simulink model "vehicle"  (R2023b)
settings: Solver=ode3  StartTime=0.0  StopTime=t_end  FixedStep=dt8dof  RelTol=1e-3
PreLoadFcn:
  | define_swarm_buses(3, 1000);
model workspace (MAT data in the model file):
  Af = 1.8
  Cp_tyre = 500
  Cx = 0.28
  G = 15000
  Ha = 0.4
  Hg = 0.4
  Hroll = 0.304
  Hroll_f = 0.08
  Hroll_r = 0.12
  Ir = 0.8
  Ix = 450
  Jz = 1800
  K = 130000
  K_psi = 0.48
  K_y = 0.06
  Karb_F = 26000
  Karb_R = 26000
  KdF = 0
  KdR = 0
  Kd_h = 0
  Kd_v = 0
  Kd_y = 0
  Ki_h = 0
  Ki_v = 0.1
  Ki_y = 0
  Kp_h = 1.5
  Kp_v = 1.5
  Kp_y = 0.1
  Ks_f = 39000
  Ks_r = 39000
  Kv = 290000
  L = 1.5
  Lril_L = 0.055
  Lril_T = 0.5
  MAX_PATH_LEN = 1000
  Pacn = [3000 1 1 1 1 1 1 1 1 0 0 0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]
  R0 = 0.2
  Rfront = 0.2
  Rr_sterzo = 0
  Rrear = 0.2
  Rs = 13
  Tf = 1.5
  Tr = 1.5
  a = 0.6
  a_brake = -3
  b = 0.9
  camb_0F = 0
  camb_0R = -0.00680678408278
  d_max = 0.558505360638
  dt8dof = 0.002
  dtastar = 0.1
  dtcontrol = 0.03
  f0 = 0.0041
  f2 = 2.051e-07
  g = 9.81
  m = 1300
  mot_T_table = [0 0 0 0 0 0 0 0 0 0 0 0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]
  mot_alpha_bp = [0 10 20 30 40 50 60 70 80 90 100]
  mot_n_bp = [0 29.9163426864 59.8326853729 89.7490280593 119.665370746 149.581713432 179.498056119 209.414398805 239.330741492 269.247084178 299.163426864 329.079769551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]
  mpc_speed : object (value not decoded)
  phi_road0 = 0
  psi0 = 0
  r_goal = 5
  r_slow = 30
  replan_steps = 20
  rho = 1.3
  slope_x_body0 = 0
  slope_y_body0 = 0
  t_end = 70
  terrain_truth_mu_table = [-1 -1 -1 -1 -1 -1 -1 -1 -1 -1 -1 -1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]
  terrain_truth_obstacle_table = [1 1 1 1 1 1 1 1 1 1 1 1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]
  terrain_truth_slope_deg_table = [2.67415653197 2.67413215857 2.67406695826 2.6739952249 2.6739164067 2.67382991742 2.67373513563 2.67363140411 2.67351802953 2.67339428225 2.67325939642 2.67311257041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]
  terrain_truth_slope_x_table = [-0.0458815772305 -0.0458808922252 -0.0458794511544 -0.0458778616187 -0.0458761104845 -0.0458741837099 -0.0458720663111 -0.0458697423295 -0.0458671948025 -0.0458644057365 -0.0458613560839 -0.045858025724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]
  terrain_truth_slope_y_table = [0.00874081815183 0.00874213563744 0.00874360556 0.00874524373283 0.00874706738108 0.00874909524079 0.00875134766185 0.00875384671474 0.00875661630067 0.00875968226488 0.00876307251276 0.0087668171283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]
  terrain_truth_traversable_table = [0 0 0 0 0 0 0 0 0 0 0 0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]
  terrain_truth_x_bp = [0 1 2 3 4 5 6 7 8 9 10 11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]
  terrain_truth_y_bp = [0 1 2 3 4 5 6 7 8 9 10 11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]
  teta0 = 0
  tetapunto0 = 0
  theta_road0 = 0
  toe_F = -0.00174532925199
  toe_R = 0.00174532925199
  velstart = 5
  wr0_FL = 3.15
  wr0_FR = 3.15
  wr0_RL = 3.15
  wr0_RR = 3.15
  x0 = 0
  y0 = 0
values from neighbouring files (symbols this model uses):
  gear_ratio = 10    [motor_map.m]
  v_ref_init = scenario.vehicle8.velstart    [make_vref_filter.m]
undefined symbols (not defined in the file or in its folder): A_f, B_f, C_f, D_f, psi0_1
libraries: simulink_extras x15, mpclib x1, slpidlib x1
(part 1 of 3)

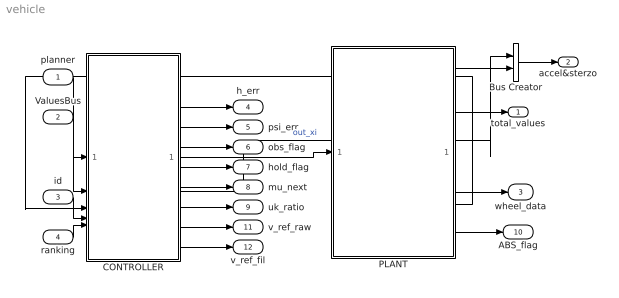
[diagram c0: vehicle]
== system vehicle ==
  planner : Inport  OutDataTypeStr=Bus: PlannerPath  SampleTime=.1
  ValuesBus : Inport  Port=2  OutDataTypeStr=Bus: ValuesBus
  id : Inport  Port=3
  ranking : Inport  Port=4  PortDimensions=3
  Bus Creator : BusCreator  Inputs=2  OutDataTypeStr=Bus: AccelSterzo
  CONTROLLER : Subsystem
  PLANT : Subsystem
  total_values : Outport  OutDataTypeStr=Bus: VehicleState
  accel&sterzo : Outport  Port=2  OutDataTypeStr=Bus: AccelSterzo
  wheel_data : Outport  Port=3  OutDataTypeStr=Bus: WheelData
  h_err : Outport  Port=4
  psi_err : Outport  Port=5
  obs_flag : Outport  Port=6
  hold_flag : Outport  Port=7
  mu_next : Outport  Port=8
  uk_ratio : Outport  Port=9
  ABS_flag : Outport  Port=10
  v_ref_raw : Outport  Port=11
  v_ref_fil : Outport  Port=12
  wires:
  PLANT/1(Out_delta) -> Bus Creator/2
  CONTROLLER/2(Out_xi) -> Bus Creator/1  "out_xi"
  planner/1 -> CONTROLLER/1(from planner)
  CONTROLLER/1(to_plant) -> PLANT/1(from_controller)
  Bus Creator/1 -> accel&sterzo/1
  PLANT/2(total_values) -> total_values/1
  PLANT/3(to_controller) -> CONTROLLER/3(from_plant)
  id/1 -> CONTROLLER/4(id)
  ranking/1 -> CONTROLLER/5(ranking)
  ValuesBus/1 -> CONTROLLER/2(ValuesBus)
  PLANT/4(wheel_data) -> wheel_data/1
  CONTROLLER/3(e_cte) -> h_err/1
  CONTROLLER/4(psi_e) -> psi_err/1
  CONTROLLER/5(obs_flag) -> obs_flag/1
  CONTROLLER/6(hold_flag) -> hold_flag/1
  CONTROLLER/7(mu next) -> mu_next/1
  CONTROLLER/8(unk_ratio) -> uk_ratio/1
  PLANT/5(ABS_flag) -> ABS_flag/1
  CONTROLLER/9(v_ref_raw) -> v_ref_raw/1
  CONTROLLER/10(v_ref_fil) -> v_ref_fil/1

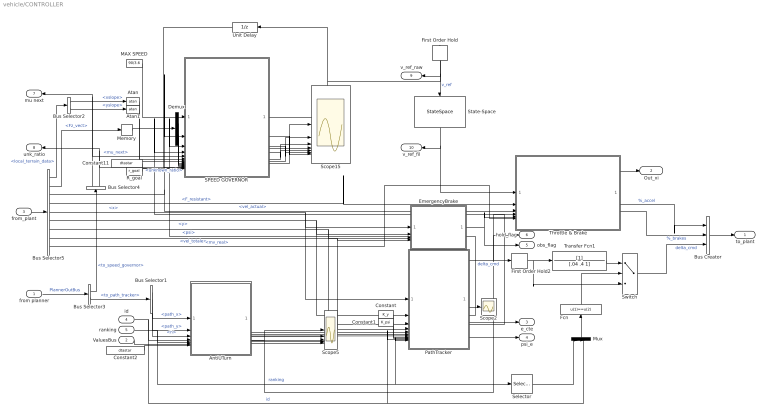
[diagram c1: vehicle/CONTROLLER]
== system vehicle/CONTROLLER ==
  from planner : Inport
  ValuesBus : Inport  Port=2
  from_plant : Inport  Port=3
  id : Inport  Port=4
  ranking : Inport  Port=5
  AntiUTurn : MATLAB Function  TreatAsAtomicUnit=on
  Atan : Trigonometry  Operator=atan
  Atan1 : Trigonometry  Operator=atan
  Bus Creator : BusCreator  Inputs=3
  Bus Selector1 : BusSelector  OutputSignals=path_x,path_y,n
  Bus Selector2 : BusSelector  OutputSignals=slope_vehicle.xslope,slope_vehicle.yslope
  Bus Selector3 : BusSelector  OutputSignals=to_speed_governor,to_path_tracker
  Bus Selector4 : BusSelector  OutputSignals=mu_next,unknown_ratio
  Bus Selector5 : BusSelector  OutputSignals=local_terrain_data,Fz_vect,vel_actual,F_resistant,signal2.x,signal2.y,signal2.psi,signal2.vel_totale,mv_real
  Constant : Constant  Value=K_y
  Constant1 : Constant  Value=K_psi
  Constant11 : Constant  Value=dtastar
  Constant2 : Constant  Value=dtastar
  Demux : Demux
  EmergencyBrake : MATLAB Function  TreatAsAtomicUnit=on
  Fcn : Fcn  Expr=u(1)==u(2)
  First Order Hold : FirstOrderHold  InitialOutput=v_ref_init  ErrorTolerance=inf
  First Order Hold2 : FirstOrderHold  ErrorTolerance=inf
  MAX SPEED : Constant  Value=90/3.6
  Memory : Memory
  Mux : Mux  Inputs=2
  PathTracker : MATLAB Function  TreatAsAtomicUnit=on
  R_goal : Constant  Value=r_goal
  SPEED GOVERNOR : MATLAB Function  TreatAsAtomicUnit=on
  Scope15 : Scope  NumInputPorts=7
  Scope2 : Scope
  Scope5 : Scope  NumInputPorts=5
  Selector : Selector  InputPortWidth=3  IndexOptions=Index vector (dialog)  Indices=[1]  OutputSizes=1
  State-Space : StateSpace  A=A_f  B=B_f  C=C_f  D=D_f  InitialCondition=v_ref_init
  Switch : Switch  Criteria=u2 > Threshold
  Throttle & Brake : Subsystem
  Transfer Fcn1 : TransferFcn  Denominator=[.04 .4 1]
  Unit Delay : UnitDelay  InitialCondition=velstart  SampleTime=-1  HasFrameUpgradeWarning=on
  to_plant : Outport
  Out_xi : Outport  Port=2
  e_cte : Outport  Port=3
  psi_e : Outport  Port=4
  obs_flag : Outport  Port=5
  hold_flag : Outport  Port=6
  mu next : Outport  Port=7
  unk_ratio : Outport  Port=8
  v_ref_raw : Outport  Port=9
  v_ref_fil : Outport  Port=10
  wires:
  Constant11/1 -> SPEED GOVERNOR/14(Ts)
  PathTracker/6(psi_e) -> psi_e/1
  PathTracker/3(dist_to_goal) -> SPEED GOVERNOR/4(d_goal)
  MAX SPEED/1 -> SPEED GOVERNOR/1("v_max_global ")
  Bus Selector4/1 -> SPEED GOVERNOR/5(mu_next), mu next/1  "<mu_next>"
  SPEED GOVERNOR/2(v_ref_raw) -> Scope15/1
  Bus Selector3/1 -> Bus Selector4/1  "<to_speed_governor>"
  from planner/1 -> Bus Selector3/1  "PlannerOutBus"
  PathTracker/2(kappa_next) -> SPEED GOVERNOR/3(kappa_next)
  Bus Selector5/6 -> PathTracker/2(y), EmergencyBrake/2(y)  "<y>"
  PathTracker/1(delta_cmd) -> First Order Hold2/1  "delta_cmd"
  Bus Selector5/5 -> PathTracker/1(x), EmergencyBrake/1(x)  "<x>"
  Bus Selector5/7 -> PathTracker/3(psi), EmergencyBrake/3(psi)  "<psi>"
  SPEED GOVERNOR/7(v_unknown) -> Scope15/6
  PathTracker/4(goal_flag) -> Scope2/1
  SPEED GOVERNOR/8(v_ltr) -> Scope15/7
  First Order Hold/1 -> State-Space/1, v_ref_raw/1  "v_ref"
  SPEED GOVERNOR/4(v_curve_mu) -> Scope15/3
  Bus Selector2/2 -> Atan1/1  "<yslope>"
  SPEED GOVERNOR/1(v_ref) -> First Order Hold/1, Unit Delay/1
  Memory/1 -> Demux/1
  Atan1/1 -> SPEED GOVERNOR/7(angle_lat)
  SPEED GOVERNOR/3(v_max_global) -> Scope15/2
  Bus Selector2/1 -> Atan/1  "<xslope>"
  Demux/3 -> SPEED GOVERNOR/10(Fz_RL)
  SPEED GOVERNOR/6(v_goal) -> Scope15/5
  Bus Selector4/2 -> SPEED GOVERNOR/12(unknown_ratio_ahead), unk_ratio/1  "<unknown_ratio>"
  SPEED GOVERNOR/5(v_rollover) -> Scope15/4
  Atan/1 -> SPEED GOVERNOR/6(angle_long)
  Demux/1 -> SPEED GOVERNOR/8(Fz_FL)
  Bus Selector3/2 -> Bus Selector1/1  "<to_path_tracker>"
  Demux/2 -> SPEED GOVERNOR/9(Fz_FR)
  R_goal/1 -> SPEED GOVERNOR/15(r_goal)
  Demux/4 -> SPEED GOVERNOR/11(Fz_RR)
  Constant/1 -> PathTracker/8(K_y)
  Constant1/1 -> PathTracker/9(K_psi)
  Bus Creator/1 -> to_plant/1
  from_plant/1 -> Bus Selector5/1
  Bus Selector5/3 -> SPEED GOVERNOR/2(V), Throttle & Brake/3(v_actual)  "<vel_actual>"
  Bus Selector5/1 -> Bus Selector2/1  "<local_terrain_data>"
  Bus Selector5/2 -> Memory/1  "<Fz_vect>"
  Throttle & Brake/2(% accel) -> Bus Creator/1  "%_accel"
  Throttle & Brake/3(brakes) -> Bus Creator/2  "%_brakes"
  Throttle & Brake/1(Out_xi) -> Out_xi/1
  Bus Selector5/4 -> Throttle & Brake/2(F_res)  "<F_resistant>"
  Bus Selector5/8 -> PathTracker/4(vel), EmergencyBrake/4(vel)  "<vel_totale>"
  First Order Hold2/1 -> Transfer Fcn1/1, Switch/3
  AntiUTurn/1(path_x_out) -> PathTracker/5(path_x)
  AntiUTurn/2(path_y_out) -> PathTracker/6(path_y)
  AntiUTurn/3(n_out) -> PathTracker/7(n_pts)
  Bus Selector1/1 -> AntiUTurn/1(path_x_in)  "<path_x>"
  Bus Selector1/2 -> AntiUTurn/2(path_y_in)  "<path_y>"
  Bus Selector1/3 -> AntiUTurn/3(n_in)  "<n>"
  id/1 -> AntiUTurn/4(id), Mux/2, PathTracker/10(id)  "id"
  ranking/1 -> Selector/1, PathTracker/11(ranking), AntiUTurn/5(ranking)  "ranking"
  ValuesBus/1 -> AntiUTurn/6(ValuesBus)
  Constant2/1 -> AntiUTurn/7(Ts)
  AntiUTurn/4(hold_flag) -> Scope5/1, hold_flag/1, Throttle & Brake/4(hold_flag)
  AntiUTurn/5(allow_uturn) -> Scope5/2
  AntiUTurn/6(long_rel) -> Scope5/3
  AntiUTurn/7(wait_s) -> Scope5/4
  AntiUTurn/8(mode) -> Scope5/5
  EmergencyBrake/1(obs_flag) -> obs_flag/1, Throttle & Brake/5(emergency_flag)
  Unit Delay/1 -> SPEED GOVERNOR/13(v_ref_prev)
  State-Space/1 -> Throttle & Brake/1(v_ref), v_ref_fil/1
  PathTracker/5(e_cte) -> e_cte/1
  Switch/1 -> Bus Creator/3  "delta_cmd"
  Selector/1 -> Mux/1
  Mux/1 -> Fcn/1
  Fcn/1 -> Switch/2
  Transfer Fcn1/1 -> Switch/1
  Bus Selector5/9 -> Throttle & Brake/6(mv_real)  "<mv_real>"

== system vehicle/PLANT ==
  note: questi sono i plot degli slip, far vedere come si notano i diversi sample time: ogni .1 cambia il comando motore e lo slip torna ad oscillare, ma grazie alle lunghezze di rilassamento (che rendono stiff il problema) lo slip si smorza intorno al valore
  from_controller : Inport
  Bus Creator : BusCreator  Inputs=6
  Bus Selector : BusSelector  OutputSignals=delta_cmd,%_accel,%_brakes
  ENGINE : Subsystem
  Gain : Gain  Gain=-1
  Rate Limiter delta : RateLimiter  RisingSlewLimit=1.5  FallingSlewLimit=-1.5  SampleTimeMode=inherited
  Sat_delta : Saturate  UpperLimit=d_max  LowerLimit=-d_max
  VEHICLE 8DOF : Subsystem
  get_values : Subsystem
  Out_delta : Outport
  total_values : Outport  Port=2
  to_controller : Outport  Port=3
  wheel_data : Outport  Port=4
  ABS_flag : Outport  Port=5
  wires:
  get_values/3(local terrain data) -> Bus Creator/6, VEHICLE 8DOF/4(terrain)  "local_terrain_data"
  VEHICLE 8DOF/3(speed_vel) -> get_values/1(speed_vel)
  get_values/1(total_values) -> total_values/1, Bus Creator/2
  ENGINE/1(Cm_vect) -> VEHICLE 8DOF/2(Cm_vect)
  Rate Limiter delta/1 -> Out_delta/1, VEHICLE 8DOF/1(delta)  "delta_sterzo"
  Sat_delta/1 -> Rate Limiter delta/1
  get_values/2(vel_actual) -> Bus Creator/3  "vel_actual"
  Gain/1 -> Sat_delta/1
  VEHICLE 8DOF/2(Fz_vect) -> Bus Creator/1  "Fz_vect"
  from_controller/1 -> Bus Selector/1
  Bus Selector/1 -> Gain/1  "<delta_cmd>"
  Bus Creator/1 -> to_controller/1
  Bus Selector/2 -> ENGINE/2(% accel)  "<%_accel>"
  Bus Selector/3 -> VEHICLE 8DOF/3(%brakes)  "<%_brakes>"
  VEHICLE 8DOF/4(F_res) -> Bus Creator/4  "F_resistant"
  VEHICLE 8DOF/1(wheel_data) -> wheel_data/1, ENGINE/1(wheel_data)
  VEHICLE 8DOF/5(ABS_flag) -> ABS_flag/1
  VEHICLE 8DOF/6(mv_real) -> Bus Creator/5  "mv_real"

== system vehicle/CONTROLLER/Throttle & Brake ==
  v_ref : Inport
  F_res : Inport  Port=2
  v_actual : Inport  Port=3
  hold_flag : Inport  Port=4
  emergency_flag : Inport  Port=5
  mv_real : Inport  Port=6
  Abs : Abs
  Add : Sum
  Const_zero_alpha : Constant  Value=0
  Constant : Constant  Value=0
  Constant1 : Constant  Value=-400
  MATLAB Function : MATLAB Function  TreatAsAtomicUnit=on
  MPC Controller : mpclib/MPC Controller  SCDEnableBlockLinearizationSpecification=on  mpcobj=mpc_speed  is_multiple=0  enable_value=0  return_u0=off  updateMPCinCallerWorkspace=on  md_inport=on  mv_inport=on  uref_inport=off  return_cost=off  return_mvseq=off  return_qpstatus=off  return_xseq=off  return_state=off  return_ovseq=off  state_inport=off  umin_inport=off  umax_inport=off  ymin_inport=off  ymax_inport=on  cc_inport=off  ywt_inport=off  uwt_inport=off  duwt_inport=off  rhoeps_inport=off  pm_inport=off  MaximumP=20  HorizonChoice=FixedHorizon  n_ts=0.03  n_p=30  n_mv=1  n_md=1  n_ud=0  n_mo=1  n_uo=0  BlockDataType=double  SampleTimeInherited=off  switch_inport=off
  Max_alpha_pos : MinMax  Function=max  Inputs=2
  Min : MinMax  Inputs=2
  Switch : Switch  Criteria=u2 > Threshold
  Switch1 : Switch  Criteria=u2 > Threshold
  Switch2 : Switch  Criteria=u2 > Threshold
  Unit Delay : UnitDelay  SampleTime=-1  HasFrameUpgradeWarning=on
  Zero-Order Hold : ZeroOrderHold  SampleTime=dt8dof
  Out_xi : Outport
  % accel : Outport  Port=2
  brakes : Outport  Port=3
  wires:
  Zero-Order Hold/1 -> Min/1, Max_alpha_pos/1
  v_ref/1 -> MPC Controller/2, MPC Controller/5
  v_actual/1 -> MPC Controller/1, MATLAB Function/1(v_actual)
  Max_alpha_pos/1 -> Switch/3  "% accel"
  Const_zero_alpha/1 -> Min/2, Max_alpha_pos/2
  hold_flag/1 -> Add/2
  Constant/1 -> Switch/1
  Switch/1 -> Switch2/2, Switch2/1, % accel/1
  Add/1 -> Switch/2
  emergency_flag/1 -> Switch1/2, Add/1
  Constant1/1 -> Switch1/1
  Min/1 -> Switch1/3
  Switch1/1 -> Switch2/3, Abs/1
  Switch2/1 -> Unit Delay/1, Out_xi/1
  Abs/1 -> brakes/1
  MPC Controller/1 -> Zero-Order Hold/1
  F_res/1 -> MATLAB Function/3(F_res)
  Unit Delay/1 -> MATLAB Function/2(accel_prev)
  MATLAB Function/1(F_md) -> MPC Controller/3
  mv_real/1 -> MPC Controller/4

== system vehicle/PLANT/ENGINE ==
  wheel_data : Inport
  % accel : Inport  Port=2
  Apply_factor : Product  Inputs=**
  Bus Selector1 : BusSelector  OutputSignals=w_r_vect,slip_vect
  Gain_gear : Gain  Gain=gear_ratio
  Gain_n2 : Gain  Gain=gear_ratio*60/(2*pi)
  Motor_Map4 : Lookup_n-D  BreakpointsForDimension1=mot_n_bp  BreakpointsForDimension2=mot_alpha_bp  BreakpointsForDimension3=[5, 7]  Table=mot_T_table  ExtrapMethod=Clip  InternalRulePriority=Speed  RndMeth=Simplest
  TC_PI : slpidlib/PID Controller  Controller=PI  Form=Parallel  TimeDomain=Continuous-time  UseExternalTs=off  SampleTime=-1  IntegratorMethod=Forward Euler  FilterMethod=Forward Euler  ControllerParametersSource=internal  P=4  I=15  UseKiTs=off  D=0  N=100  UseFilter=on  TunerSelectOption=Transfer Function Based (PID Tuner App)  InitialConditionSource=internal  InitialConditionForIntegrator=1  InitialConditionForFilter=0  DifferentiatorICPrevScaledInput=0  ExternalReset=none  TrackingMode=off  Kt=1  LimitOutput=on  SatLimitsSource=internal  UpperSaturationLimit=1  LowerSaturationLimit=0  LinearizeAsGain=on  AntiWindupMode=clamping  Kb=1  LimitIntegrator=off  UpperIntegratorSaturationLimit=inf  LowerIntegratorSaturationLimit=-inf  POutMin=[]  POutMax=[]  IOutMin=[]  IOutMax=[]  DOutMin=[]  DOutMax=[]  NOutMin=[]  NOutMax=[]  SumOutMin=[]  SumOutMax=[]  SaturationOutMin=[]  SaturationOutMax=[]  PParamMin=[]  PParamMax=[]  IParamMin=[]  IParamMax=[]  DParamMin=[]  DParamMax=[]  NParamMin=[]  NParamMax=[]  KbParamMin=[]  KbParamMax=[]  KtParamMin=[]  KtParamMax=[]  KbOutMin=[]  KbOutMax=[]  KtOutMin=[]  KtOutMax=[]  IntegratorOutMin=[]  IntegratorOutMax=[]  FilterOutMin=[]  FilterOutMax=[]  SumI1OutMin=[]  SumI1OutMax=[]  SumI2OutMin=[]  SumI2OutMax=[]  SumI3OutMin=[]  SumI3OutMax=[]  SumI4OutMin=[]  SumI4OutMax=[]  SumDOutMin=[]  SumDOutMax=[]  DifferentiatorOutMin=[]  DifferentiatorOutMax=[]  FilterDiffOutCoefMin=[]  FilterDiffOutCoefMax=[]  ReciprocalOutMin=[]  ReciprocalOutMax=[]  SumDenOutMin=[]  SumDenOutMax=[]  SumNumOutMin=[]  SumNumOutMax=[]  DivideOutMin=[]  DivideOutMax=[]  UdiffTsProdOutMin=[]  UdiffTsProdOutMax=[]  NTsProdOutMin=[]  NTsProdOutMax=[]  UintegralTsProdOutMin=[]  UintegralTsProdOutMax=[]  UngainTsProdOutMin=[]  UngainTsProdOutMax=[]  ClampingZeroOutDataTypeStr=Inherit: Inherit via back propagation  ClampingZeroOutMin=[]  ClampingZeroOutMax=[]  FilterDenConstantOutDataTypeStr=Inherit: Inherit via back propagation  FilterDenConstantOutMin=[]  FilterDenConstantOutMax=[]  PCopyOutDataTypeStr=Inherit: Inherit via back propagation  PCopyOutMin=[]  PCopyOutMax=[]  NCopyOutDataTypeStr=Inherit: Inherit via back propagation  NCopyOutMin=[]  NCopyOutMax=[]  IntegratorContinuousStateAttributes=''  IntegratorStateMustResolveToSignalObject=off  IntegratorRTWStateStorageClass=Auto  FilterContinuousStateAttributes=''  FilterStateMustResolveToSignalObject=off  FilterRTWStateStorageClass=Auto  ParallelPVariant=InternalParameters  IdealPVariant=Disabled  IVariant=InternalParameters  DVariant=Disabled  IntegratorVariant=Continuous  SatVariant=Enabled  AWVariant=ContClampingParallel  PCopyVariant=Disabled  TRVariant=Disabled  FdbkBlocksVariant=Forward  IdealPFdbkVariant=Disabled  SatFdbkVariant=Disabled  DerivativeFilterVariant=Disabled  NVariant=Disabled  NCopyVariant=Disabled_SignalSpec  FilterICVariant=Disabled  IntegratorICVariant=InternalICs  ExternalResetVariant=Disabled  TRSumVariant=Passthrough  SumFdbkVariant=Disabled  SumVariant=Sum_PI  TsampFilterVariant=InternalTs  TsampNgainVariant=Passthrough  TsampIntegralVariant=Disabled_SignalSpec  ExternalSaturationOutDataTypeStr=Inherit: Same as second input
  alpha_sat : Saturate  UpperLimit=100  LowerLimit=0
  sigma_star : Constant  Value=0.10
  slip_err : Sum  Inputs=+-
  Cm_vect : Outport
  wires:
  wheel_data/1 -> Bus Selector1/1
  alpha_sat/1 -> Motor_Map4/2
  TC_PI/1 -> Apply_factor/2
  sigma_star/1 -> slip_err/1
  Apply_factor/1 -> alpha_sat/1
  Bus Selector1/1 -> Gain_n2/1  "<w_r_vect>"
  Bus Selector1/2 -> slip_err/2  "<slip_vect>"
  Gain_gear/1 -> Cm_vect/1
  slip_err/1 -> TC_PI/1
  Gain_n2/1 -> Motor_Map4/1
  Motor_Map4/1 -> Gain_gear/1
  % accel/1 -> Apply_factor/1

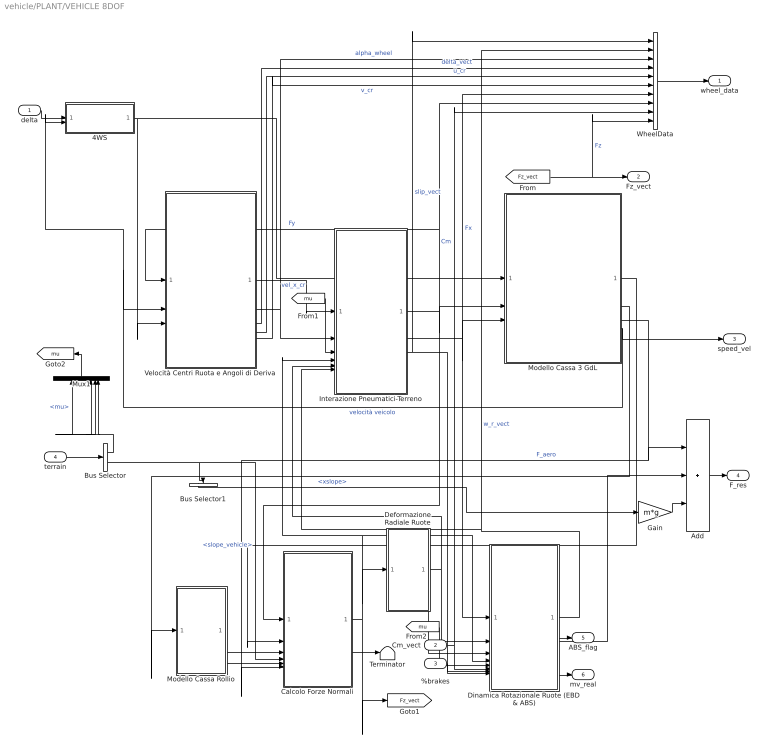
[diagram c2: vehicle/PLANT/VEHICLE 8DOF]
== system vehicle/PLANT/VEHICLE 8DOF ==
  delta : Inport
  Cm_vect : Inport  Port=2
  %brakes : Inport  Port=3
  terrain : Inport  Port=4
  4WS : Subsystem
  Add : Sum  Inputs=+++
  Bus Selector : BusSelector  OutputSignals=mu,slope_vehicle
  Bus Selector1 : BusSelector  OutputSignals=xslope
  Calcolo Forze Normali : Subsystem
  Deformazione Radiale Ruote : Subsystem
  Dinamica Rotazionale Ruote (EBD & ABS) : Subsystem
  Gain : Gain  Gain=m*g
  Interazione Pneumatici-Terreno : Subsystem
  Modello Cassa 3 GdL : Subsystem
  Modello Cassa Rollio : Subsystem
  Mux1 : Mux
  Terminator : Terminator
  Velocità Centri Ruota e Angoli di Deriva : Subsystem
  WheelData : BusCreator  Inputs=10
  wheel_data : Outport  VectorParamsAs1DForOutWhenUnconnected=off
  Fz_vect : Outport  Port=2
  speed_vel : Outport  Port=3
  F_res : Outport  Port=4  VectorParamsAs1DForOutWhenUnconnected=off
  ABS_flag : Outport  Port=5  VectorParamsAs1DForOutWhenUnconnected=off
  mv_real : Outport  Port=6  VectorParamsAs1DForOutWhenUnconnected=off
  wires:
  Interazione Pneumatici-Terreno/1(Fy) -> Calcolo Forze Normali/1(Fy), Modello Cassa 3 GdL/2(Fy), WheelData/8, Velocità Centri Ruota e Angoli di Deriva/1(Fy)  "Fy"
  [mu] -> Interazione Pneumatici-Terreno/3(mu)
  Interazione Pneumatici-Terreno/2(Fx) -> Modello Cassa 3 GdL/3(Fx), Dinamica Rotazionale Ruote (EBD & ABS)/1(Fx), WheelData/7  "Fx"
  Velocità Centri Ruota e Angoli di Deriva/2(alpha) -> Interazione Pneumatici-Terreno/2(alpha), WheelData/3  "alpha_wheel"
  Dinamica Rotazionale Ruote (EBD & ABS)/1(w_r) -> Interazione Pneumatici-Terreno/6(w_r), WheelData/2  "w_r_vect"
  Deformazione Radiale Ruote/1(Rr) -> Dinamica Rotazionale Ruote (EBD & ABS)/2(Rr), Interazione Pneumatici-Terreno/5(Rr)
  Deformazione Radiale Ruote/2(Rc) -> Dinamica Rotazionale Ruote (EBD & ABS)/3(Rc)
  Modello Cassa 3 GdL/3(F_aero) -> Calcolo Forze Normali/6(Faero), Add/1  "F_aero"
  Calcolo Forze Normali/2("FzF/FzR ") -> Terminator/1
  %brakes/1 -> Dinamica Rotazionale Ruote (EBD & ABS)/7(%brakes)
  Mux1/1 -> [mu]
  Modello Cassa 3 GdL/2(a_y) -> Modello Cassa Rollio/1(acc_y)
  Cm_vect/1 -> Dinamica Rotazionale Ruote (EBD & ABS)/6(Cm), WheelData/9  "Cm"
  Velocità Centri Ruota e Angoli di Deriva/1(vel_x_cr) -> Interazione Pneumatici-Terreno/1(vel_x_cr)  "vel_x_cr"
  Modello Cassa Rollio/1(phi_punto) -> Calcolo Forze Normali/3(phi_punto)
  Modello Cassa 3 GdL/1(a_x) -> Calcolo Forze Normali/2(acc_x)
  Modello Cassa Rollio/2(phi) -> Calcolo Forze Normali/5(phi)
  Interazione Pneumatici-Terreno/3(slip_vector) -> Dinamica Rotazionale Ruote (EBD & ABS)/8(slip_vect), WheelData/1  "slip_vect"
  terrain/1 -> Bus Selector/1
  Bus Selector/1 -> Mux1/1, Mux1/2, Mux1/3, Mux1/4  "<mu>"
  Bus Selector/2 -> Bus Selector1/1, Calcolo Forze Normali/4(slope)  "<slope_vehicle>"
  Modello Cassa 3 GdL/4(velocità_veicolo) -> speed_vel/1, 4WS/2(velocità_veicolo), Velocità Centri Ruota e Angoli di Deriva/2(velocità_veicolo)  "velocità veicolo"
  4WS/1(delta_ruote) -> Modello Cassa 3 GdL/1(delta_cmd), Velocità Centri Ruota e Angoli di Deriva/3(delta_cmd)
  delta/1 -> 4WS/1(delta_sterzo)
  WheelData/1 -> wheel_data/1
  Calcolo Forze Normali/1(Fz) -> Deformazione Radiale Ruote/1(Fz), Dinamica Rotazionale Ruote (EBD & ABS)/4(Fz), Interazione Pneumatici-Terreno/4(Fz), [Fz_vect]
  Dinamica Rotazionale Ruote (EBD & ABS)/2(R_roll_tot) -> Add/2
  Add/1 -> F_res/1
  Gain/1 -> Add/3
  Bus Selector1/1 -> Gain/1  "<xslope>"
  [mu] -> Dinamica Rotazionale Ruote (EBD & ABS)/5(mu)
  Velocità Centri Ruota e Angoli di Deriva/3(delta_vect) -> WheelData/4  "delta_vect"
  Velocità Centri Ruota e Angoli di Deriva/4(u_cr) -> WheelData/5  "u_cr"
  Velocità Centri Ruota e Angoli di Deriva/5(v_cr) -> WheelData/6  "v_cr"
  [Fz_vect] -> WheelData/10, Fz_vect/1  "Fz"
  Dinamica Rotazionale Ruote (EBD & ABS)/3(ABS_flag) -> ABS_flag/1
  Dinamica Rotazionale Ruote (EBD & ABS)/4(mv_real) -> mv_real/1

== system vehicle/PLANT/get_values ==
  speed_vel : Inport
  Bus Creator2 : BusCreator  Inputs=4
  Bus Selector : BusSelector  OutputSignals=uv
  Constant5 : Constant  Value=x0
  Constant6 : Constant  Value=y0
  Integrator : Integrator  InitialConditionSource=external
  Integrator1 : Integrator  InitialConditionSource=external
  Lookup Tables : Subsystem
  Pitagora : Subsystem
  rotazione : Subsystem
  total_values : Outport
  vel_actual : Outport  Port=2
  local terrain data : Outport  Port=3
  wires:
  Integrator/1 -> Lookup Tables/1(x), Bus Creator2/1  "x"
  Constant5/1 -> Integrator/2
  Constant6/1 -> Integrator1/2
  rotazione/1(x_dot) -> Integrator/1
  Integrator1/1 -> Lookup Tables/2(y), Bus Creator2/2  "y"
  rotazione/2(y_dot) -> Integrator1/1
  Pitagora/1(vel_actual) -> Bus Creator2/4, vel_actual/1  "vel_totale"
  Lookup Tables/1(data) -> local terrain data/1
  speed_vel/1 -> Bus Selector/1, rotazione/1(velocità_veicolo)
  Bus Selector/1 -> Pitagora/1(u_v)  "<uv>"
  rotazione/3(psi) -> Lookup Tables/3(psi), Bus Creator2/3  "psi"
  Bus Creator2/1 -> total_values/1

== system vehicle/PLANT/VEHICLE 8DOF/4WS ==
  delta_sterzo : Inport
  velocità_veicolo : Inport  Port=2
  100km/h : Constant  Value=28
  Bus Creator : BusCreator  Inputs=2
  Bus Selector : BusSelector  OutputSignals=uv.u
  Constant : Constant
  Divide : Product  Inputs=**
  Divide1 : Product  Inputs=*/
  Divide2 : Product  Inputs=**
  Fcn : Fcn  Expr=1/(1+exp(-(u(1)-u(2))/2.22))
  Fcn1 : Fcn  Expr=u(3)+u(1)*(u(2)-u(3))
  Gain2 : Gain  Gain=.3
  K2_high : Constant  Value=.3
  K2_low : Constant  Value=-.4
  Min : MinMax  Inputs=2
  Minus : Sum  Inputs=-+
  Mux : Mux  Inputs=2
  Mux1 : Mux  Inputs=3
  vel_transizione : Constant  Value=10
  delta_ruote : Outport
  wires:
  Divide1/1 -> Min/1
  velocità_veicolo/1 -> Bus Selector/1
  100km/h/1 -> Divide1/2
  Bus Selector/1 -> Divide1/1, Mux/1  "<u>"
  Min/1 -> Gain2/1
  vel_transizione/1 -> Mux/2
  Constant/1 -> Minus/2, Min/2
  Mux/1 -> Fcn/1
  Fcn/1 -> Mux1/1  "sigmoide"
  K2_high/1 -> Mux1/2
  K2_low/1 -> Mux1/3
  Gain2/1 -> Minus/1
  Mux1/1 -> Fcn1/1
  Minus/1 -> Divide/1  "gain_ant"
  delta_sterzo/1 -> Divide/2, Divide2/1
  Fcn1/1 -> Divide2/2  "gain_post"
  Divide/1 -> Bus Creator/1  "delta_F"
  Divide2/1 -> Bus Creator/2  "delta_R"
  Bus Creator/1 -> delta_ruote/1

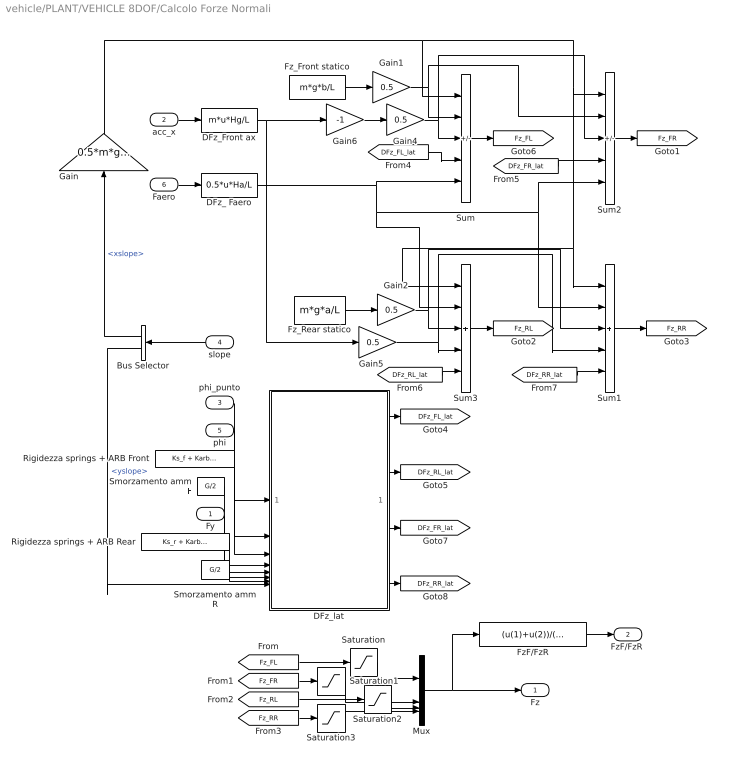
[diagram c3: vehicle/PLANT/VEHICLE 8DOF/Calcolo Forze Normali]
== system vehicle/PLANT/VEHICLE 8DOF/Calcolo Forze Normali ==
  Fy : Inport
  acc_x : Inport  Port=2
  phi_punto : Inport  Port=3
  slope : Inport  Port=4
  phi : Inport  Port=5
  Faero : Inport  Port=6
  Bus Selector : BusSelector  OutputSignals=xslope,yslope
  DFz_ Faero : Fcn  Expr=0.5*u*Ha/L
  DFz_Front ax : Fcn  Expr=m*u*Hg/L
  DFz_lat : Subsystem
  FzF/FzR : Fcn  Expr=(u(1)+u(2))/(u(3)+u(4))
  Fz_Front statico : Constant  Value=m*g*b/L
  Fz_Rear statico : Constant  Value=m*g*a/L
  Gain : Gain  Gain=0.5*m*g*Hg/L
  Gain{1..2,4..5} (4 alike) : Gain  Gain=0.5
  Gain6 : Gain  Gain=-1
  Mux : Mux
  Rigidezza springs + ARB Front : Constant  Value=Ks_f + Karb_F
  Rigidezza springs + ARB Rear : Constant  Value=Ks_r + Karb_R
  Saturation{,1..3} (4 alike) : Saturate  UpperLimit=inf  LowerLimit=0
  Smorzamento amm F : Constant  Value=G/2
  Smorzamento amm R : Constant  Value=G/2
  Sum : Sum  Inputs=-+++-
  Sum1 : Sum  Inputs=+++++
  Sum2 : Sum  Inputs=-+++-
  Sum3 : Sum  Inputs=+++++
  Fz : Outport  VectorParamsAs1DForOutWhenUnconnected=off
  "FzF/FzR " : Outport  Port=2  VectorParamsAs1DForOutWhenUnconnected=off
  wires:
  Fz_Front statico/1 -> Gain1/1
  Sum3/1 -> [Fz_RL]
  Sum/1 -> [Fz_FL]
  Sum2/1 -> [Fz_FR]
  Sum1/1 -> [Fz_RR]
  Gain5/1 -> Sum1/4, Sum3/4
  DFz_Front ax/1 -> Gain6/1, Gain5/1
  acc_x/1 -> DFz_Front ax/1
  phi_punto/1 -> DFz_lat/1(phipunto)
  phi/1 -> DFz_lat/2(phi)
  Rigidezza springs + ARB Front/1 -> DFz_lat/3(K_f)
  Smorzamento amm F/1 -> DFz_lat/4(C_f)
  Gain2/1 -> Sum1/3, Sum3/3
  Fz_Rear statico/1 -> Gain2/1
  Gain1/1 -> Sum/2, Sum2/2
  Gain4/1 -> Sum/3, Sum2/3
  Gain6/1 -> Gain4/1
  [Fz_FL] -> Saturation/1
  [Fz_FR] -> Saturation1/1
  [Fz_RL] -> Saturation2/1
  [Fz_RR] -> Saturation3/1
  Fy/1 -> DFz_lat/5(Fy)
  Rigidezza springs + ARB Rear/1 -> DFz_lat/6(K_r)
  Saturation/1 -> Mux/1
  Saturation1/1 -> Mux/2
  Saturation2/1 -> Mux/3
  Saturation3/1 -> Mux/4
  Mux/1 -> FzF/FzR/1, Fz/1
  Faero/1 -> DFz_ Faero/1
  DFz_ Faero/1 -> Sum3/2, Sum2/5, Sum1/2, Sum/5
  FzF/FzR/1 -> "FzF/FzR "/1
  Smorzamento amm R/1 -> DFz_lat/7(C_r)
  DFz_lat/1(DFz_FL_lat) -> [DFz_FL_lat]
  [DFz_FL_lat] -> Sum/4
  DFz_lat/2(DFz_RL_lat) -> [DFz_RL_lat]
  DFz_lat/3(DFz_FR_lat) -> [DFz_FR_lat]
  DFz_lat/4(DFz_RR_lat) -> [DFz_RR_lat]
  [DFz_FR_lat] -> Sum2/4
  [DFz_RL_lat] -> Sum3/5
  [DFz_RR_lat] -> Sum1/5
  slope/1 -> Bus Selector/1
  Bus Selector/2 -> DFz_lat/8(slope)  "<yslope>"
  Gain/1 -> Sum2/1, Sum3/1, Sum1/1, Sum/1
  Bus Selector/1 -> Gain/1  "<xslope>"

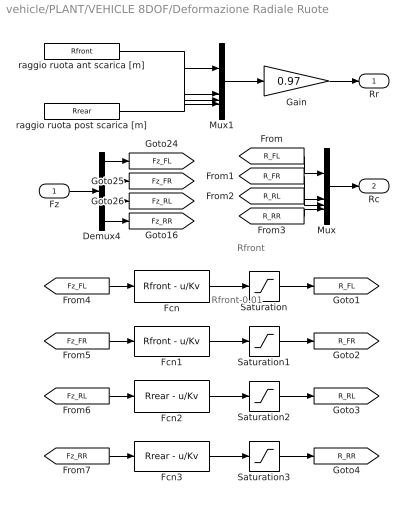
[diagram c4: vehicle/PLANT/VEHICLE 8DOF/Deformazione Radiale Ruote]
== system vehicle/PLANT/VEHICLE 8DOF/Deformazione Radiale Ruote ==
  note: Rfront-0.01
  note: Rfront
  Fz : Inport
  Demux4 : Demux
  Fcn : Fcn  Expr=Rfront - u/Kv
  Fcn1 : Fcn  Expr=Rfront - u/Kv
  Fcn2 : Fcn  Expr=Rrear - u/Kv
  Fcn3 : Fcn  Expr=Rrear - u/Kv
  Gain : Gain  Gain=0.97
  Mux : Mux
  Mux1 : Mux
  Saturation : Saturate  UpperLimit=Rfront  LowerLimit=Rfront-0.01
  Saturation1 : Saturate  UpperLimit=Rfront  LowerLimit=Rfront-0.01
  Saturation2 : Saturate  UpperLimit=Rrear  LowerLimit=Rrear-0.01
  Saturation3 : Saturate  UpperLimit=Rrear  LowerLimit=Rrear-0.01
  raggio ruota ant scarica [m] : Constant  Value=Rfront
  raggio ruota post scarica [m] : Constant  Value=Rrear
  Rr : Outport  VectorParamsAs1DForOutWhenUnconnected=off
  Rc : Outport  Port=2  VectorParamsAs1DForOutWhenUnconnected=off
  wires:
  Fcn3/1 -> Saturation3/1
  [Fz_RR] -> Fcn3/1
  Fcn2/1 -> Saturation2/1
  [Fz_RL] -> Fcn2/1
  Fcn1/1 -> Saturation1/1
  Fcn/1 -> Saturation/1
  [Fz_FL] -> Fcn/1
  [R_FL] -> Mux/1
  [R_FR] -> Mux/2
  [R_RL] -> Mux/3
  [R_RR] -> Mux/4
  Mux/1 -> Rc/1
  [Fz_FR] -> Fcn1/1
  Fz/1 -> Demux4/1
  Demux4/1 -> [Fz_FL]
  Demux4/2 -> [Fz_FR]
  Demux4/3 -> [Fz_RL]
  Demux4/4 -> [Fz_RR]
  Saturation/1 -> [R_FL]
  Saturation1/1 -> [R_FR]
  Saturation2/1 -> [R_RL]
  Saturation3/1 -> [R_RR]
  raggio ruota post scarica [m]/1 -> Mux1/3, Mux1/4
  raggio ruota ant scarica [m]/1 -> Mux1/2, Mux1/1
  Mux1/1 -> Gain/1
  Gain/1 -> Rr/1

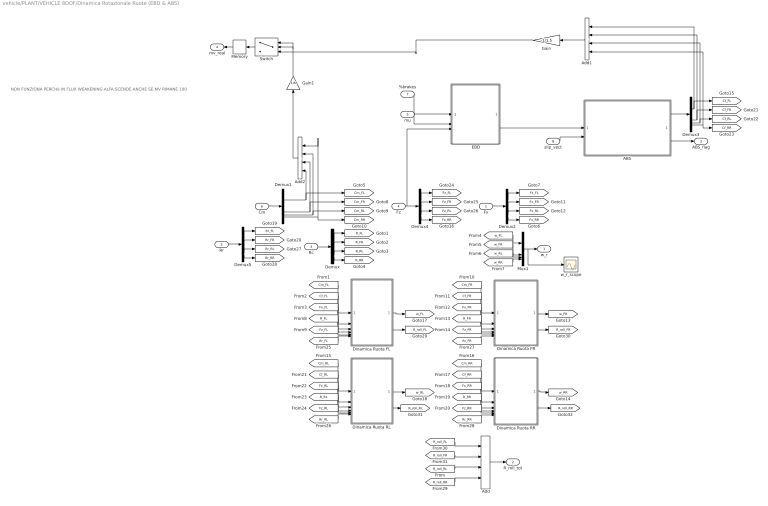
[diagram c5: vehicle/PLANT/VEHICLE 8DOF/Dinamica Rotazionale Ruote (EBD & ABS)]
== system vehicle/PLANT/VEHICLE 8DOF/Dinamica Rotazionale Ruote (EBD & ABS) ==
  note: NON FUNZIONA PERCHé IN FLUX WEAKENING ALFA SCENDE ANCHE SE MV RIMANE 100
  Fx : Inport
  Rr : Inport  Port=2
  Rc : Inport  Port=3
  Fz : Inport  Port=4
  mu : Inport  Port=5
  Cm : Inport  Port=6
  %brakes : Inport  Port=7
  slip_vect : Inport  Port=8
  ABS : Subsystem
  Add : Sum  Inputs=++++
  Add1 : Sum  Inputs=++++
  Add2 : Sum  Inputs=++++
  Demux{,1..5} (6 alike) : Demux
  Dinamica Ruota FL : Subsystem
  Dinamica Ruota FR : Subsystem
  Dinamica Ruota RL : Subsystem
  Dinamica Ruota RR : Subsystem
  EBD : Subsystem
  Gain : Gain  Gain=-1/1.5
  Gain1 : Gain  Gain=1/6
  Memory : Memory
  Mux1 : Mux
  Switch : Switch  Criteria=u2 > Threshold
  w_r_scope : Scope
  w_r : Outport  VectorParamsAs1DForOutWhenUnconnected=off
  R_roll_tot : Outport  Port=2
  ABS_flag : Outport  Port=3
  mv_real : Outport  Port=4
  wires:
  Dinamica Ruota FL/1(w) -> [w_FL]
  Rc/1 -> Demux/1
  Demux/1 -> [R_FL]
  Demux/2 -> [R_FR]
  Demux/3 -> [R_RL]
  Demux/4 -> [R_RR]
  Cm/1 -> Demux1/1
  Demux1/1 -> Add2/4, [Cm_FL]
  Demux1/2 -> Add2/3, [Cm_FR]
  Demux1/3 -> Add2/2, [Cm_RL]
  Demux1/4 -> Add2/1, [Cm_RR]
  Demux3/1 -> [Cf_FL], Add1/1
  Demux3/2 -> [Cf_FR], Add1/2
  Demux3/3 -> [Cf_RL], Add1/3
  Demux3/4 -> [Cf_RR], Add1/4
  Fz/1 -> EBD/3(Fz), Demux4/1
  Demux4/1 -> [Fz_FL]
  Demux4/2 -> [Fz_FR]
  Demux4/3 -> [Fz_RL]
  Demux4/4 -> [Fz_RR]
  Fx/1 -> Demux2/1
  Demux2/1 -> [Fx_FL]
  Demux2/2 -> [Fx_FR]
  Demux2/3 -> [Fx_RL]
  Demux2/4 -> [Fx_RR]
  [Cm_FL] -> Dinamica Ruota FL/1(Cm)
  [Cf_FL] -> Dinamica Ruota FL/2(%brakes)
  [Fx_FL] -> Dinamica Ruota FL/3(Fx)
  [R_FL] -> Dinamica Ruota FL/4(R)
  [Fz_FL] -> Dinamica Ruota FL/5(Fz)
  Dinamica Ruota FR/1(w) -> [w_FR]
  [Cm_FR] -> Dinamica Ruota FR/1(Cm)
  [Cf_FR] -> Dinamica Ruota FR/2(Cf)
  [Fx_FR] -> Dinamica Ruota FR/3(Fx)
  [R_FR] -> Dinamica Ruota FR/4(R)
  [Fz_FR] -> Dinamica Ruota FR/5(Fz)
  Dinamica Ruota RL/1(w) -> [w_RL]
  [Cm_RL] -> Dinamica Ruota RL/1(Cm)
  [Cf_RL] -> Dinamica Ruota RL/2(Cf)
  [Fx_RL] -> Dinamica Ruota RL/3(Fx)
  [R_RL] -> Dinamica Ruota RL/4(R)
  [Fz_RL] -> Dinamica Ruota RL/5(Fz)
  [Cm_RR] -> Dinamica Ruota RR/1(Cm)
  [Cf_RR] -> Dinamica Ruota RR/2(Cf)
  [Fx_RR] -> Dinamica Ruota RR/3(Fx)
  [R_RR] -> Dinamica Ruota RR/4(R)
  [Fz_RR] -> Dinamica Ruota RR/5(Fz)
  Dinamica Ruota RR/1(w) -> [w_RR]
  [w_FL] -> Mux1/1
  [w_FR] -> Mux1/2
  [w_RL] -> Mux1/3
  [w_RR] -> Mux1/4
  Mux1/1 -> w_r_scope/1, w_r/1
  Rr/1 -> Demux5/1
  Demux5/4 -> [Rr_RR]
  Demux5/3 -> [Rr_RL]
  Demux5/2 -> [Rr_FR]
  Demux5/1 -> [Rr_FL]
  [Rr_FL] -> Dinamica Ruota FL/6(Rr)
  [Rr_RL] -> Dinamica Ruota RL/6(Rr)
  [Rr_FR] -> Dinamica Ruota FR/6(Rr)
  [Rr_RR] -> Dinamica Ruota RR/6(Rr)
  Dinamica Ruota FL/2(R_roll) -> [R_roll_FL]
  Dinamica Ruota FR/2(R_roll) -> [R_roll_FR]
  Dinamica Ruota RL/2(R_roll) -> [R_roll_RL]
  Dinamica Ruota RR/2(R_roll) -> [R_roll_RR]
  [R_roll_RR] -> Add/4
  [R_roll_RL] -> Add/3
  [R_roll_FR] -> Add/2
  [R_roll_FL] -> Add/1
  Add/1 -> R_roll_tot/1
  EBD/1(Cf) -> ABS/1(brakes_in)
  mu/1 -> EBD/2(mu)
  ABS/1(brakes_out) -> Demux3/1
  slip_vect/1 -> ABS/2(slip)
  ABS/2(flag) -> ABS_flag/1
  Add1/1 -> Gain/1
  Add2/1 -> Gain1/1
  Gain1/1 -> Switch/2, Switch/1
  Gain/1 -> Switch/3
  Switch/1 -> Memory/1
  Memory/1 -> mv_real/1
  %brakes/1 -> EBD/1(%brake)

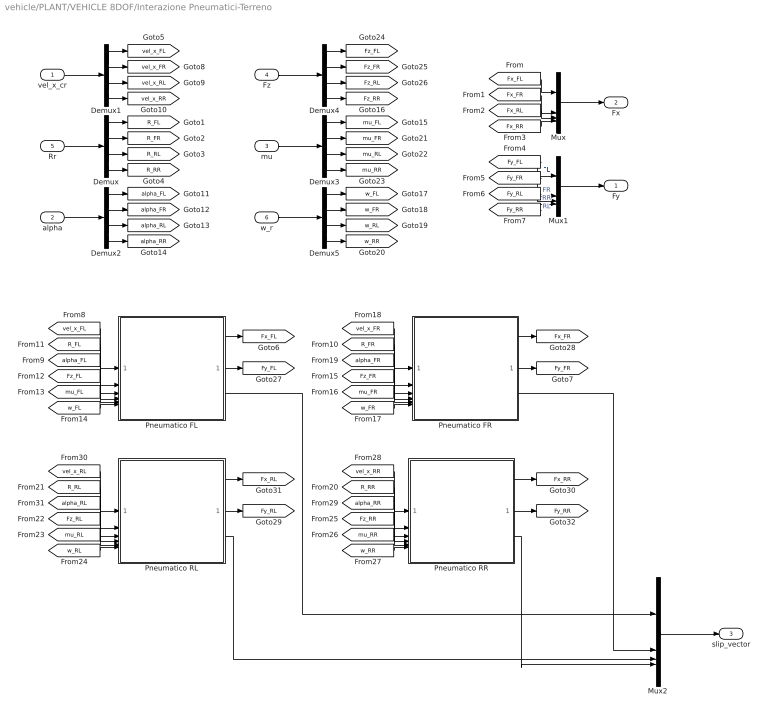
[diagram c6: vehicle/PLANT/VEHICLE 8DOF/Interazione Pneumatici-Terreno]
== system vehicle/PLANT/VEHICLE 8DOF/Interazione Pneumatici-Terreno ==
  vel_x_cr : Inport
  alpha : Inport  Port=2
  mu : Inport  Port=3
  Fz : Inport  Port=4
  Rr : Inport  Port=5
  w_r : Inport  Port=6
  Demux{,1..5} (6 alike) : Demux
  Mux : Mux
  Mux1 : Mux
  Mux2 : Mux
  Pneumatico FL : Subsystem
  Pneumatico FR : Subsystem
  Pneumatico RL : Subsystem
  Pneumatico RR : Subsystem
  Fy : Outport  VectorParamsAs1DForOutWhenUnconnected=off
  Fx : Outport  Port=2  VectorParamsAs1DForOutWhenUnconnected=off
  slip_vector : Outport  Port=3
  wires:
  [vel_x_FL] -> Pneumatico FL/1(vel_x)
  [R_FL] -> Pneumatico FL/2(R)
  [alpha_FL] -> Pneumatico FL/3(alfa)
  [Fz_FL] -> Pneumatico FL/4(Fz)
  [mu_FL] -> Pneumatico FL/5(mu_strada)
  Pneumatico FL/1(Fx_rit) -> [Fx_FL]
  Pneumatico FL/2(Fy_rit) -> [Fy_FL]
  [w_FL] -> Pneumatico FL/6(w)
  [Fx_FL] -> Mux/1
  [Fx_FR] -> Mux/2
  [Fx_RL] -> Mux/3
  [Fx_RR] -> Mux/4
  [Fy_FL] -> Mux1/1  "FL"
  [Fy_FR] -> Mux1/2  "FR"
  [Fy_RL] -> Mux1/3  "RL"
  [Fy_RR] -> Mux1/4  "RR"
  Rr/1 -> Demux/1
  Demux/1 -> [R_FL]
  Demux/2 -> [R_FR]
  Demux/3 -> [R_RL]
  Demux/4 -> [R_RR]
  vel_x_cr/1 -> Demux1/1
  Demux1/1 -> [vel_x_FL]
  Demux1/2 -> [vel_x_FR]
  Demux1/3 -> [vel_x_RL]
  Demux1/4 -> [vel_x_RR]
  alpha/1 -> Demux2/1
  Demux2/1 -> [alpha_FL]
  Demux2/2 -> [alpha_FR]
  Demux2/3 -> [alpha_RL]
  Demux2/4 -> [alpha_RR]
  mu/1 -> Demux3/1
  Demux3/1 -> [mu_FL]
  Demux3/2 -> [mu_FR]
  Demux3/3 -> [mu_RL]
  Demux3/4 -> [mu_RR]
  Demux4/1 -> [Fz_FL]
  Demux4/2 -> [Fz_FR]
  Demux4/3 -> [Fz_RL]
  Demux4/4 -> [Fz_RR]
  w_r/1 -> Demux5/1
  Demux5/1 -> [w_FL]
  Demux5/2 -> [w_FR]
  Demux5/3 -> [w_RL]
  Demux5/4 -> [w_RR]
  [vel_x_FR] -> Pneumatico FR/1(vel_x)
  [R_FR] -> Pneumatico FR/2(R)
  [alpha_FR] -> Pneumatico FR/3(alfa)
  [Fz_FR] -> Pneumatico FR/4(Fz)
  [mu_FR] -> Pneumatico FR/5(mu_strada)
  Pneumatico FR/1(Fx_rit) -> [Fx_FR]
  Pneumatico FR/2(Fy_rit) -> [Fy_FR]
  [w_FR] -> Pneumatico FR/6(w)
  [vel_x_RL] -> Pneumatico RL/1(vel_x)
  [R_RL] -> Pneumatico RL/2(R)
  [alpha_RL] -> Pneumatico RL/3(alfa)
  [Fz_RL] -> Pneumatico RL/4(Fz)
  [mu_RL] -> Pneumatico RL/5(mu_strada)
  Pneumatico RL/1(Fx_rit) -> [Fx_RL]
  Pneumatico RL/2(Fy_rit) -> [Fy_RL]
  [w_RL] -> Pneumatico RL/6(w)
  [vel_x_RR] -> Pneumatico RR/1(vel_x)
  [R_RR] -> Pneumatico RR/2(R)
  [alpha_RR] -> Pneumatico RR/3(alfa)
  [Fz_RR] -> Pneumatico RR/4(Fz)
  [mu_RR] -> Pneumatico RR/5(mu_strada)
  Pneumatico RR/1(Fx_rit) -> [Fx_RR]
  Pneumatico RR/2(Fy_rit) -> [Fy_RR]
  [w_RR] -> Pneumatico RR/6(w)
  Fz/1 -> Demux4/1
  Mux2/1 -> slip_vector/1
  Mux/1 -> Fx/1
  Mux1/1 -> Fy/1
  Pneumatico FL/3(slip_FL) -> Mux2/1
  Pneumatico FR/3(slip_FR) -> Mux2/2
  Pneumatico RL/3(slip_RL) -> Mux2/3
  Pneumatico RR/3(slip_RR) -> Mux2/4

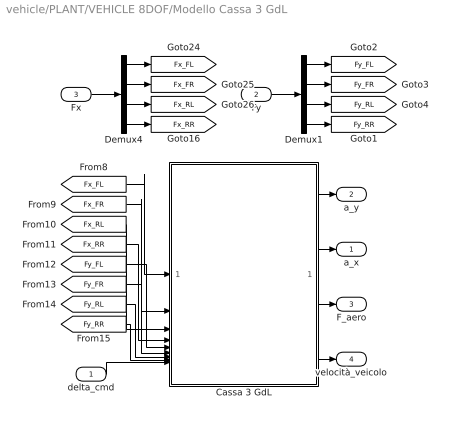
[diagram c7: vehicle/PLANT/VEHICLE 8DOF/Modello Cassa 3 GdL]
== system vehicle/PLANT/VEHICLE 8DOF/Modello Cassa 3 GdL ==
  delta_cmd : Inport
  Fy : Inport  Port=2
  Fx : Inport  Port=3
  Cassa 3 GdL : Subsystem
  Demux1 : Demux
  Demux4 : Demux
  a_x : Outport  VectorParamsAs1DForOutWhenUnconnected=off
  a_y : Outport  Port=2  VectorParamsAs1DForOutWhenUnconnected=off
  F_aero : Outport  Port=3  VectorParamsAs1DForOutWhenUnconnected=off
  velocità_veicolo : Outport  Port=4
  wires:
  Fx/1 -> Demux4/1
  Demux4/1 -> [Fx_FL]
  Demux4/2 -> [Fx_FR]
  Demux4/3 -> [Fx_RL]
  Demux4/4 -> [Fx_RR]
  Fy/1 -> Demux1/1
  Demux1/1 -> [Fy_FL]
  Demux1/2 -> [Fy_FR]
  Demux1/3 -> [Fy_RL]
  Demux1/4 -> [Fy_RR]
  Cassa 3 GdL/1(a_y) -> a_y/1
  Cassa 3 GdL/2(a_x) -> a_x/1
  [Fx_FL] -> Cassa 3 GdL/1(Fx_FL)
  [Fx_FR] -> Cassa 3 GdL/2(Fx_FR)
  [Fx_RL] -> Cassa 3 GdL/3(Fx_RL)
  [Fx_RR] -> Cassa 3 GdL/4(Fx_RR)
  [Fy_FL] -> Cassa 3 GdL/5(Fy_FL)
  [Fy_FR] -> Cassa 3 GdL/6(Fy_FR)
  [Fy_RL] -> Cassa 3 GdL/7(Fy_RL)
  [Fy_RR] -> Cassa 3 GdL/8(Fy_RR)
  delta_cmd/1 -> Cassa 3 GdL/9(Delta)
  Cassa 3 GdL/3(F_aero) -> F_aero/1
  Cassa 3 GdL/4(velocità_veicolo) -> velocità_veicolo/1

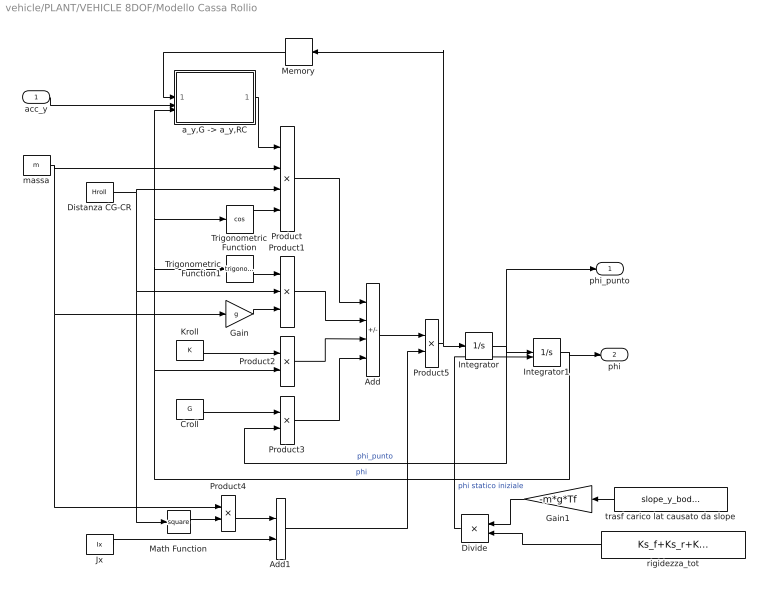
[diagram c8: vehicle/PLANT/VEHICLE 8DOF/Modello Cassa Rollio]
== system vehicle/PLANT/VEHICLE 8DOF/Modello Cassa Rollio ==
  acc_y : Inport
  Add : Sum  Inputs=++--
  Add1 : Sum
  Croll : Constant  Value=G
  Distanza CG-CR : Constant  Value=Hroll
  Divide : Product  Inputs=*/
  Gain : Gain  Gain=g
  Gain1 : Gain  Gain=-m*g*Tf
  Integrator : Integrator
  Integrator1 : Integrator  InitialConditionSource=external
  Jx : Constant  Value=Ix
  Kroll : Constant  Value=K
  Math Function : Math  Operator=square  SignedPower=on
  Memory : Memory
  Product : Product  Inputs=4  RndMeth=Zero
  Product1 : Product  Inputs=3  RndMeth=Zero
  Product2 : Product  RndMeth=Zero
  Product3 : Product  RndMeth=Zero
  Product4 : Product  RndMeth=Zero
  Product5 : Product  Inputs=*/  RndMeth=Zero
  Trigonometric Function : Trigonometry  Operator=cos
  Trigonometric Function1 : Trigonometry
  "a_y,G -> a_y,RC" : Subsystem
  massa : Constant  Value=m
  rigidezza_tot : Constant  Value=Ks_f+Ks_r+Karb_F+Karb_R
  trasf carico lat causato da slope : Constant  Value=slope_y_body0
  phi_punto : Outport  VectorParamsAs1DForOutWhenUnconnected=off
  phi : Outport  Port=2  VectorParamsAs1DForOutWhenUnconnected=off
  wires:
  massa/1 -> Product/2, Gain/1, Product4/1
  acc_y/1 -> "a_y,G -> a_y,RC"/2(a_y,G)
  Distanza CG-CR/1 -> Math Function/1, Product1/2, Product/3
  Trigonometric Function/1 -> Product/4
  Product/1 -> Add/1
  Product1/1 -> Add/2
  Product2/1 -> Add/3
  Product3/1 -> Add/4
  Croll/1 -> Product3/1
  Kroll/1 -> Product2/1
  Integrator/1 -> phi_punto/1, Integrator1/1, Product3/2  "phi_punto"
  Integrator1/1 -> phi/1, Trigonometric Function1/1, Trigonometric Function/1, "a_y,G -> a_y,RC"/3("teta "), Product2/2  "phi"
  Add1/1 -> Product5/2
  Product5/1 -> Integrator/1, Memory/1
  Add/1 -> Product5/1
  Product4/1 -> Add1/1
  Math Function/1 -> Product4/2
  Jx/1 -> Add1/2
  Gain/1 -> Product1/3
  Trigonometric Function1/1 -> Product1/1
  Memory/1 -> "a_y,G -> a_y,RC"/1(teta_pp)
  "a_y,G -> a_y,RC"/1(a_y,RC) -> Product/1
  rigidezza_tot/1 -> Divide/2
  trasf carico lat causato da slope/1 -> Gain1/1
  Divide/1 -> Integrator1/2  "phi statico iniziale"
  Gain1/1 -> Divide/1

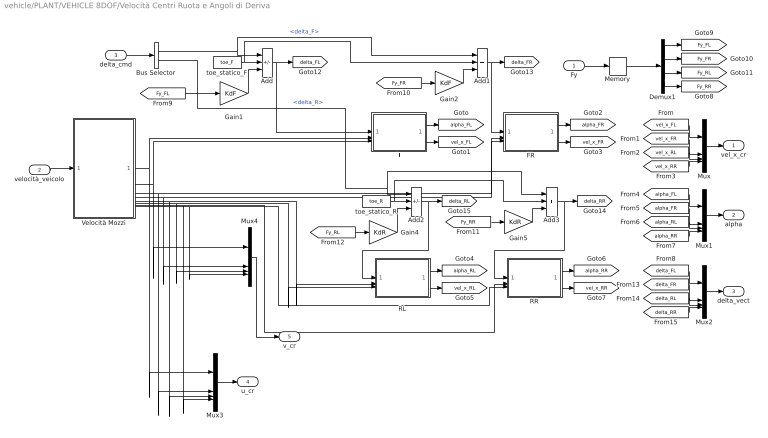
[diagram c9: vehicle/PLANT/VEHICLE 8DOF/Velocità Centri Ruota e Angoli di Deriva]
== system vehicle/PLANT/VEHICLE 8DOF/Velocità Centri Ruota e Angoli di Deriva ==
  Fy : Inport
  velocità_veicolo : Inport  Port=2
  delta_cmd : Inport  Port=3
  Add : Sum  Inputs=+-+
  Add1 : Sum  Inputs=+++
  Add2 : Sum  Inputs=+-+
  Add3 : Sum  Inputs=+++
  Bus Selector : BusSelector  OutputSignals=delta_F,delta_R
  Demux1 : Demux
  FL : Subsystem
  FR : Subsystem
  Gain1 : Gain  Gain=KdF  SaturateOnIntegerOverflow=on
  Gain2 : Gain  Gain=KdF  SaturateOnIntegerOverflow=on
  Gain4 : Gain  Gain=KdR  SaturateOnIntegerOverflow=on
  Gain5 : Gain  Gain=KdR  SaturateOnIntegerOverflow=on
  Memory : Memory
  Mux{,1..4} (5 alike) : Mux
  RL : Subsystem
  RR : Subsystem
  Velocità Mozzi : Subsystem
  toe_statico_F : Constant  Value=toe_F
  toe_statico_R : Constant  Value=toe_R
  vel_x_cr : Outport  VectorParamsAs1DForOutWhenUnconnected=off
  alpha : Outport  Port=2  VectorParamsAs1DForOutWhenUnconnected=off
  delta_vect : Outport  Port=3  VectorParamsAs1DForOutWhenUnconnected=off
  u_cr : Outport  Port=4  VectorParamsAs1DForOutWhenUnconnected=off
  v_cr : Outport  Port=5  VectorParamsAs1DForOutWhenUnconnected=off
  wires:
  RL/2(vel_x_cr) -> [vel_x_RL]
  RL/1(alfa) -> [alpha_RL]
  RR/2(vel_x_cr) -> [vel_x_RR]
  RR/1(alfa) -> [alpha_RR]
  FR/2(vel_x_cr) -> [vel_x_FR]
  FR/1(alfa) -> [alpha_FR]
  FL/1(alfa) -> [alpha_FL]
  FL/2(vel_x_cr) -> [vel_x_FL]
  Velocità Mozzi/8(v_RR) -> Mux4/4, RR/3(v_cr)
  Velocità Mozzi/7(u_RR) -> Mux3/4, RR/2(u_cr)
  Velocità Mozzi/6(v_RL) -> Mux4/3, RL/3(v_cr)
  Velocità Mozzi/5(u _RL) -> Mux3/3, RL/2(u_cr)
  Velocità Mozzi/4(v_FR) -> Mux4/2, FR/3(v_cr)
  Velocità Mozzi/3(u_FR) -> Mux3/2, FR/2(u_cr)
  Velocità Mozzi/2("v_FL ") -> Mux4/1, FL/3(v_cr)
  Velocità Mozzi/1("u_FL ") -> Mux3/1, FL/2(u_cr)
  [vel_x_FL] -> Mux/1
  [vel_x_FR] -> Mux/2
  [vel_x_RL] -> Mux/3
  [vel_x_RR] -> Mux/4
  Mux/1 -> vel_x_cr/1
  [alpha_FL] -> Mux1/1
  [alpha_FR] -> Mux1/2
  [alpha_RL] -> Mux1/3
  [alpha_RR] -> Mux1/4
  Mux1/1 -> alpha/1
  Bus Selector/1 -> Add/1, Add1/1  "<delta_F>"
  toe_statico_F/1 -> Add/2, Add1/2
  Add/1 -> [delta_FL], FL/1(delta)
  Add1/1 -> [delta_FR], FR/1(delta)
  Gain1/1 -> Add/3
  Fy/1 -> Memory/1
  Demux1/1 -> [Fy_FL]
  Demux1/2 -> [Fy_FR]
  Demux1/3 -> [Fy_RL]
  Demux1/4 -> [Fy_RR]
  [Fy_FL] -> Gain1/1
  Gain2/1 -> Add1/3
  [Fy_FR] -> Gain2/1
  toe_statico_R/1 -> Add2/2, Add3/2
  Add2/1 -> [delta_RL], RL/1(delta)
  Add3/1 -> [delta_RR], RR/1(delta)
  Gain4/1 -> Add2/3
  [Fy_RL] -> Gain4/1
  Gain5/1 -> Add3/3
  [Fy_RR] -> Gain5/1
  Memory/1 -> Demux1/1
  velocità_veicolo/1 -> Velocità Mozzi/1(velocità_veicolo)
  delta_cmd/1 -> Bus Selector/1
  Bus Selector/2 -> Add2/1, Add3/1  "<delta_R>"
  [delta_FR] -> Mux2/2
  [delta_RL] -> Mux2/3
  [delta_RR] -> Mux2/4
  [delta_FL] -> Mux2/1
  Mux2/1 -> delta_vect/1
  Mux3/1 -> u_cr/1
  Mux4/1 -> v_cr/1

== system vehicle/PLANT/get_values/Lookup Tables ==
  x : Inport
  y : Inport  Port=2
  psi : Inport  Port=3
  Bus Creator : BusCreator  Inputs=2
  Bus Creator1 : BusCreator  Inputs=2
  Constant13 : Constant  Value=terrain_truth_slope_x_table
  Constant14 : Constant  Value=terrain_truth_y_bp
  Constant15 : Constant  Value=terrain_truth_slope_y_table
  Constant2 : Constant  Value=terrain_truth_x_bp
  Constant3 : Constant  Value=terrain_truth_mu_table
  mu Lookup Table : Lookup_n-D  BreakpointsForDimension1Source=Input port  BreakpointsForDimension1=[1:3]  BreakpointsForDimension2Source=Input port  BreakpointsForDimension2=[1:3]  TableSource=Input port  InternalRulePriority=Speed  RndMeth=Simplest
  rotazione : Subsystem
  x slope Lookup Table : Lookup_n-D  BreakpointsForDimension1Source=Input port  BreakpointsForDimension1=[1:3]  BreakpointsForDimension2Source=Input port  BreakpointsForDimension2=[1:3]  TableSource=Input port  InternalRulePriority=Speed  RndMeth=Simplest
  y slope Lookup Table : Lookup_n-D  BreakpointsForDimension1Source=Input port  BreakpointsForDimension1=[1:3]  BreakpointsForDimension2Source=Input port  BreakpointsForDimension2=[1:3]  TableSource=Input port  InternalRulePriority=Speed  RndMeth=Simplest
  data : Outport
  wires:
  x/1 -> mu Lookup Table/2, y slope Lookup Table/2, x slope Lookup Table/2
  Constant14/1 -> x slope Lookup Table/4, y slope Lookup Table/4, mu Lookup Table/4
  Constant3/1 -> mu Lookup Table/3
  y/1 -> y slope Lookup Table/1, x slope Lookup Table/1, mu Lookup Table/1
  Constant15/1 -> y slope Lookup Table/3
  Constant13/1 -> x slope Lookup Table/3
  Constant2/1 -> y slope Lookup Table/5, x slope Lookup Table/5, mu Lookup Table/5
  x slope Lookup Table/1 -> rotazione/1(slope xabs)
  y slope Lookup Table/1 -> rotazione/2(slope yabs)
  Bus Creator/1 -> data/1
  psi/1 -> rotazione/3(-psi)
  rotazione/1(slope x vehicle) -> Bus Creator1/1  "xslope"
  rotazione/2(slope y vehicle) -> Bus Creator1/2  "yslope"
  mu Lookup Table/1 -> Bus Creator/1  "mu"
  Bus Creator1/1 -> Bus Creator/2  "slope_vehicle"

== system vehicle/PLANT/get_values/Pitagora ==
  u_v : Inport
  Bus Selector : BusSelector  OutputSignals=u,v
  Minus2 : Sum
  Square : Math  Operator=square
  Square Root : Sqrt
  Square1 : Math  Operator=square
  vel_actual : Outport
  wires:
  Minus2/1 -> Square Root/1
  Square1/1 -> Minus2/2
  Square/1 -> Minus2/1
  Square Root/1 -> vel_actual/1
  Bus Selector/1 -> Square/1  "<u>"
  Bus Selector/2 -> Square1/1  "<v>"
  u_v/1 -> Bus Selector/1

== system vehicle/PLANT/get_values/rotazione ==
  velocità_veicolo : Inport
  Bus Selector : BusSelector  OutputSignals=uv.u,uv.v,psi_punto
  Constant4 : Constant  Value=psi0
  Cos : Trigonometry  Operator=cos
  Int_psi1 : Integrator  InitialConditionSource=external  InitialCondition=psi0_1
  Minus1 : Sum
  Minus3 : Sum  Inputs=+-
  Product{,1..3} (4 alike) : Product
  Sin : Trigonometry
  x_dot : Outport
  y_dot : Outport  Port=2
  psi : Outport  Port=3
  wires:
  Product2/1 -> Minus1/1
  Product3/1 -> Minus1/2
  Cos/1 -> Product3/1, Product/2
  Sin/1 -> Product2/2, Product1/2
  Product1/1 -> Minus3/2
  Product/1 -> Minus3/1
  Minus3/1 -> x_dot/1  "x_dot"
  Minus1/1 -> y_dot/1  "y_dot"
  Int_psi1/1 -> psi/1, Sin/1, Cos/1
  velocità_veicolo/1 -> Bus Selector/1
  Constant4/1 -> Int_psi1/2
  Bus Selector/1 -> Product/1, Product2/1  "<u>"
  Bus Selector/2 -> Product3/2, Product1/1  "<v>"
  Bus Selector/3 -> Int_psi1/1  "<psi_punto>"

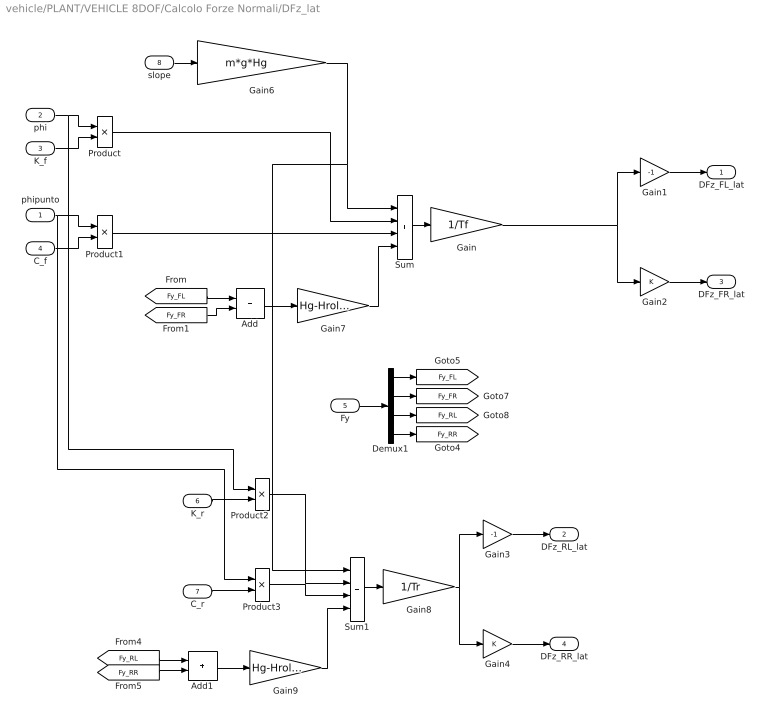
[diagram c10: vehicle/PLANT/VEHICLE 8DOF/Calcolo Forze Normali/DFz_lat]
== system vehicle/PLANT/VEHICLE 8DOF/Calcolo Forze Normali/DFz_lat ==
  phipunto : Inport
  phi : Inport  Port=2
  K_f : Inport  Port=3
  C_f : Inport  Port=4
  Fy : Inport  Port=5
  K_r : Inport  Port=6
  C_r : Inport  Port=7
  slope : Inport  Port=8
  Add : Sum
  Add1 : Sum
  Demux1 : Demux
  Gain : Gain  Gain=1/Tf
  Gain1 : Gain  Gain=-1
  Gain2 : Gain
  Gain3 : Gain  Gain=-1
  Gain4 : Gain
  Gain6 : Gain  Gain=m*g*Hg
  Gain7 : Gain  Gain=Hg-Hroll_f
  Gain8 : Gain  Gain=1/Tr
  Gain9 : Gain  Gain=Hg-Hroll_r
  Product{,1..3} (4 alike) : Product  RndMeth=Zero
  Sum : Sum  Inputs=++++
  Sum1 : Sum  Inputs=++++
  DFz_FL_lat : Outport  VectorParamsAs1DForOutWhenUnconnected=off
  DFz_RL_lat : Outport  Port=2  VectorParamsAs1DForOutWhenUnconnected=off
  DFz_FR_lat : Outport  Port=3  VectorParamsAs1DForOutWhenUnconnected=off
  DFz_RR_lat : Outport  Port=4  VectorParamsAs1DForOutWhenUnconnected=off
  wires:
  phi/1 -> Product2/1, Product/1
  K_f/1 -> Product/2
  C_f/1 -> Product1/2
  Product/1 -> Sum/2
  Product1/1 -> Sum/3
  Sum/1 -> Gain/1
  Gain/1 -> Gain1/1, Gain2/1
  Add/1 -> Gain7/1
  Gain7/1 -> Sum/4
  Fy/1 -> Demux1/1
  Demux1/1 -> [Fy_FL]
  Demux1/2 -> [Fy_FR]
  Demux1/3 -> [Fy_RL]
  Demux1/4 -> [Fy_RR]
  [Fy_FL] -> Add/1
  [Fy_FR] -> Add/2
  K_r/1 -> Product2/2
  phipunto/1 -> Product1/1, Product3/1
  C_r/1 -> Product3/2
  Product2/1 -> Sum1/2
  Product3/1 -> Sum1/3
  Sum1/1 -> Gain8/1
  Add1/1 -> Gain9/1
  Gain9/1 -> Sum1/4
  [Fy_RL] -> Add1/1
  [Fy_RR] -> Add1/2
  Gain8/1 -> Gain3/1, Gain4/1
  Gain3/1 -> DFz_RL_lat/1
  Gain4/1 -> DFz_RR_lat/1
  Gain1/1 -> DFz_FL_lat/1
  Gain2/1 -> DFz_FR_lat/1
  slope/1 -> Gain6/1
  Gain6/1 -> Sum1/1, Sum/1

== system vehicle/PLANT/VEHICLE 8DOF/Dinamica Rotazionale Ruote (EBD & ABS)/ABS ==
  brakes_in : Inport
  slip : Inport  Port=2
  ABS_Logic : MATLAB Function  TreatAsAtomicUnit=on
  Memory : Memory
  brakes_out : Outport
  flag : Outport  Port=2
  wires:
  brakes_in/1 -> ABS_Logic/1(brakes_in)
  slip/1 -> ABS_Logic/2(slip)
  Memory/1 -> ABS_Logic/3(last_brake)
  ABS_Logic/1(target) -> brakes_out/1, Memory/1
  ABS_Logic/2(flag) -> flag/1

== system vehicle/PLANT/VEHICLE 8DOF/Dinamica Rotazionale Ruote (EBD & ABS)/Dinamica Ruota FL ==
  Cm : Inport
  %brakes : Inport  Port=2
  Fx : Inport  Port=3
  R : Inport  Port=4
  Fz : Inport  Port=5
  Rr : Inport  Port=6
  Add : Sum  Inputs=+---
  Constant : Constant  Value=velstart
  Divide : Product  Inputs=*/
  Integrator2 : Integrator  InitialConditionSource=external  LowerSaturationLimit=0
  Manual Switch : ManualSwitch  CurrentSetting=0
  Mom Inerzia Ruota : Constant  Value=Ir
  Mux2 : Mux  Inputs=2
  Product3 : Product  RndMeth=Zero
  Product5 : Product  Inputs=*/  RndMeth=Zero
  Resistenza a Rotolmento : Fcn  Expr=u(1)*(f0+f2*u(2)^2)
  Saturation : Saturate  UpperLimit=inf  LowerLimit=0
  cond iniziale wr0 : Constant  Value=wr0_FL
  w : Outport  VectorParamsAs1DForOutWhenUnconnected=off
  R_roll : Outport  Port=2
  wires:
  Resistenza a Rotolmento/1 -> R_roll/1, Add/4
  Mux2/1 -> Resistenza a Rotolmento/1
  Integrator2/1 -> Saturation/1
  Fz/1 -> Mux2/1
  Product5/1 -> Integrator2/1
  Mom Inerzia Ruota/1 -> Product5/2
  Add/1 -> Product5/1
  Product3/1 -> Add/3
  R/1 -> Product3/2
  Fx/1 -> Product3/1
  %brakes/1 -> Add/2
  Cm/1 -> Add/1
  Rr/1 -> Divide/2
  cond iniziale wr0/1 -> Manual Switch/1
  Manual Switch/1 -> Integrator2/2
  Saturation/1 -> Mux2/2, w/1
  Constant/1 -> Divide/1
  Divide/1 -> Manual Switch/2
